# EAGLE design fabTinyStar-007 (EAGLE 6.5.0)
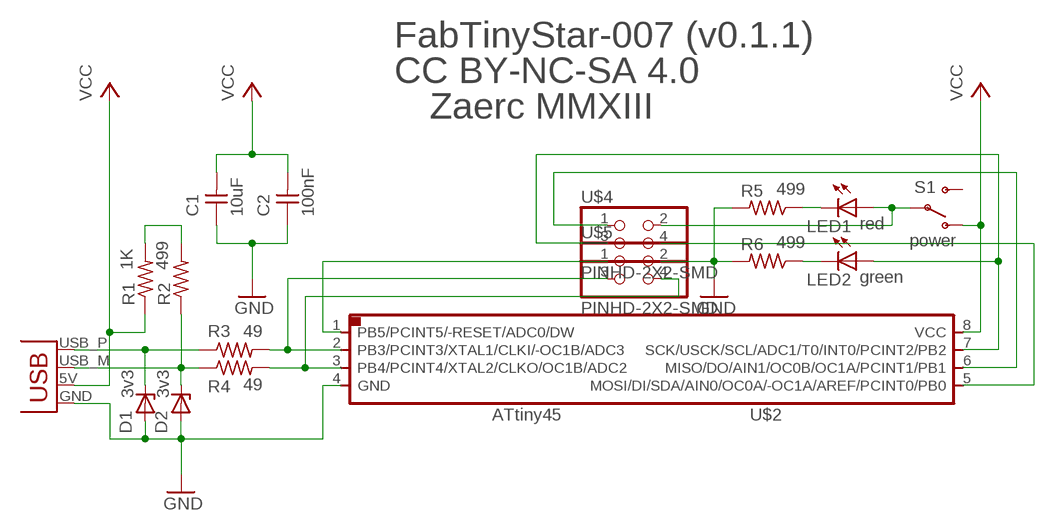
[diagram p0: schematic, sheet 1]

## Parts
C1  10uF  UNPOLARIZED_CAPACITOR1206  [1206]
C2  100nF  UNPOLARIZED_CAPACITOR1206  [1206]
D1  3v3  ZENER_DIODESOD123  [SOD123]
D2  3v3  ZENER_DIODESOD123  [SOD123]
LED1  red  LEDSMT1206  [1206]
LED2  green  LEDSMT1206  [1206]
R1  1K  RESISTOR1206  [1206]
R2  499  RESISTOR1206  [1206]
R3  49  RESISTOR1206  [1206]
R4  49  RESISTOR1206  [1206]
R5  499  RESISTOR1206  [1206]
R6  499  RESISTOR1206  [1206]
S1  power  SWITCH-SPSTSMD2  [SWITCH-SPDT-SMD]
U$1  USBPCB  [USB-A-PCB]
U$2  ATTINY45SI  [SOIC8]
U$4  PINHD-2X2-SMD  [2X02SMD]
U$5  PINHD-2X2-SMD  [2X02SMD]

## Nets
GND: C1.1 C2.1 D1.ANODE D2.ANODE R5.2 R6.2 U$1.GND U$2.4(GND) U$5.2
MISO: U$2.6(MISO/DO/AIN1/OC0B/OC1A/PCINT1/PB1) U$4.1
MOSI: U$2.5(MOSI/DI/SDA/AIN0/OC0A/-OC1A/AREF/PCINT0/PB0) U$4.4
N$1: R1.2 R2.2
N$2: R4.2 U$2.3(PB4/PCINT4/XTAL2/CLKO/OC1B/ADC2) U$5.4
N$3: D1.CATHODE R3.1 U$1.USB_P(D+)
N$4: R3.2 U$2.2(PB3/PCINT3/XTAL1/CLKI/-OC1B/ADC3) U$5.3
N$5: D2.CATHODE R2.1 R4.1 U$1.USB_M(D-)
N$13: LED2.C R6.1
N$14: LED1.C R5.1
RST: U$2.1(PB5/PCINT5/-RESET/ADC0/DW) U$5.1
SCK: LED2.A U$2.7(SCK/USCK/SCL/ADC1/T0/INT0/PCINT2/PB2) U$4.3
TVCC: LED1.A S1.2(P) U$4.2
VCC: C1.2 C2.2 R1.1 S1.1(O) U$1.5V(VBUS) U$2.8(VCC)
Unconnected: S1.3(S)

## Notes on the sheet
- FabTinyStar-007 (v0.1.1)
- CC BY-NC-SA 4.0
- Zaerc MMXIII

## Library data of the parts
C1 C2 = 01_FAB_Hello:UNPOLARIZED_CAPACITOR: unpolarized_capacitor
D1 D2 = 01_fab:ZENER_DIODE: zener diode
LED1 LED2 = led:LED: LED
R1-R6 = 01_FAB_Hello:RESISTOR
S1 = SparkFun:SWITCH-SPST: SPST Switch Simple slide switch. Spark Fun Electronics SKU : COM-00102
U$1 = SparkFun:USB: USB Connectors USB-B-PTH is fully proven SKU : PRT-00139 USB-miniB is fully proven SKU : PRT-00587 USB-A-PCB is untested. USB-A-H is throughly reviewed, but untested. Spark Fun Electronics SKU : PRT-00437 USB-B-SMT is throughly reviewed, but untested. Needs silkscreen touching up. USB-A-S has not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
U$2 = 01_fab:ATTINY45
U$4 U$5 = 01_fab:PINHD-2X2-SMD

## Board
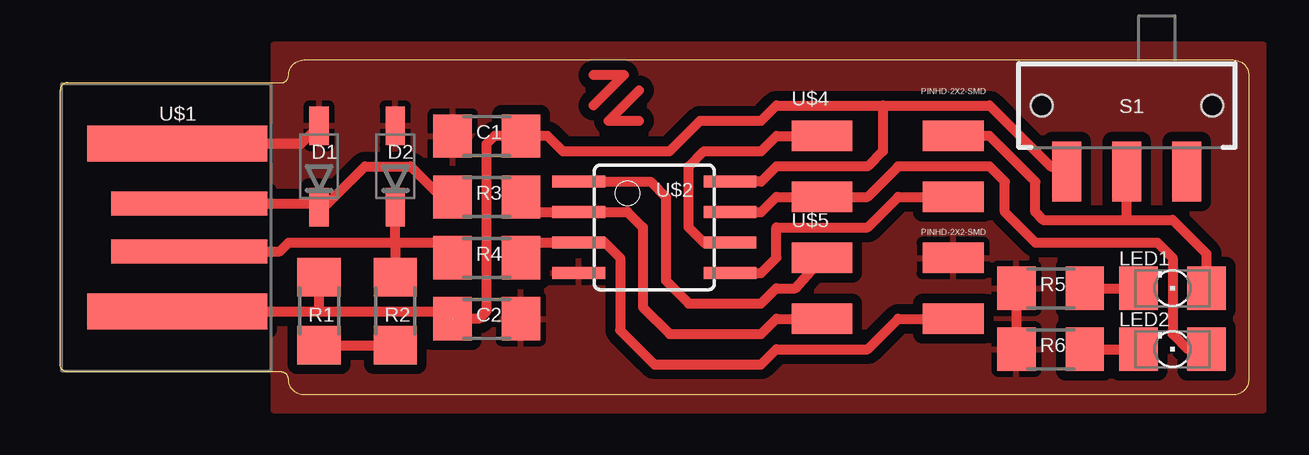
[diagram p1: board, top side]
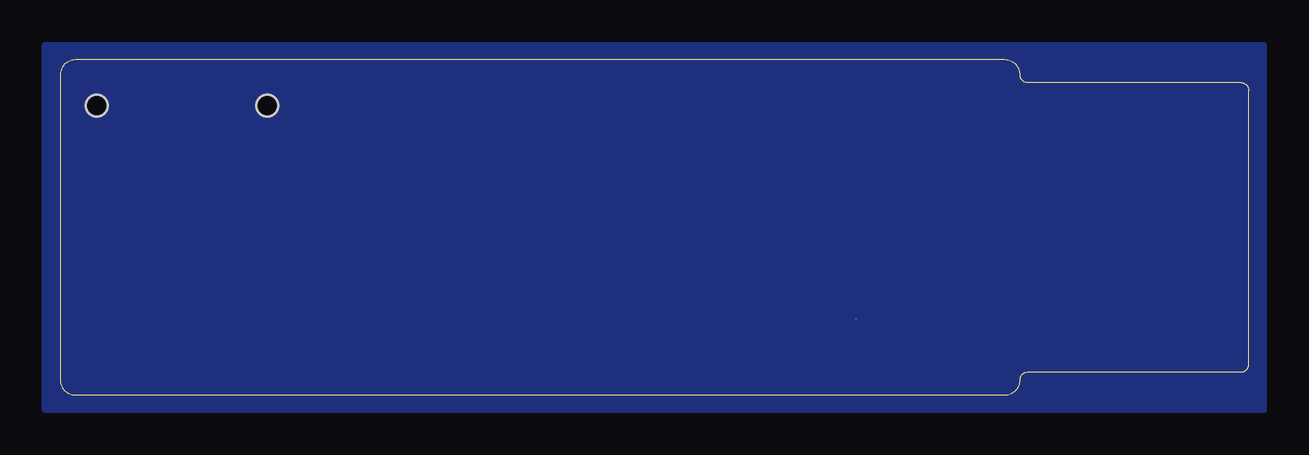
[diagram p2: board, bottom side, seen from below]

Size 49.53 x 13.97 mm. Coordinates in mm from the lower left corner, seen from the top.
Outline: 9.21,13.02 arc90 9.53,13.34 arc-90 10.16,13.97 48.9,13.97 arc-90 49.53,13.34 49.53,0.64 arc-90 48.9,0 10.16,0 arc-90 9.53,0.64 arc90 9.21,0.95 0.32,0.95 arc-90 0,1.27 0,12.7 arc-90 0.32,13.02 9.21,13.02
Copper layers (1*16): Top 0.035mm / dielectric 1.5mm / Bottom 0.035mm
Design rules "default *": minimum track width 10mil, minimum drill 24mil, track to track 16mil, track to pad 16mil, pad to pad 16mil, via to via 16mil, smd to smd 8mil, copper to edge 0mil, drill to drill 8mil, minimum pad ring 10mil, minimum via ring 8mil, stop-mask expansion 4mil, vias tented up to drill 0mil, thermal gap 10mil

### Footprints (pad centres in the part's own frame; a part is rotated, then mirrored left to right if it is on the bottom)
1206 = smd 1.6 x 1.803: 1 -1.422,0; 2 1.422,0
SOD123 = smd 1.6 x 0.8: ANODE 1.7,0; CATHODE -1.7,0
1206' = smd 1.6 x 1.803: A -1.422,0; C 1.422,0
SWITCH-SPDT-SMD = smd 1.2 x 2.5: 1 -2.5,-2.75; 2 0,-2.75; 3 2.5,-2.75 | hole 0.9: -3.55,0; 3.55,0
USB-A-PCB = smd 7.5 x 1.5: 5V -0.2,-3.5; GND -0.2,3.5 | smd 6.5 x 1: USB_M 0.3,-1; USB_P 0.3,1
SOIC8 = smd 0.5 x 2.2: 1 -1.905,-3.154; 2 -0.645,-3.154; 3 0.625,-3.154; 4 1.895,-3.154; 5 1.905,3.154; 6 0.635,3.154; 7 -0.635,3.154; 8 -1.905,3.154
2X02SMD = smd 2.54 x 1.27: 1 -2.54,1.27; 2 2.92,1.27; 3 -2.54,-1.27; 4 2.92,-1.27

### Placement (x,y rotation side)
C1  17.78,10.79 0 top
C2  17.78,3.17 180 top
D1  10.79,9.53 90 top
D2  13.97,9.53 90 top
LED1  red  [1206']  46.35,4.45 180 top
LED2  green  [1206']  46.35,1.91 180 top
R1  10.79,3.49 270 top
R2  13.97,3.49 270 top
R3  17.78,8.26 0 top
R4  17.78,5.71 0 top
R5  41.27,4.45 180 top
R6  41.27,1.91 180 top
S1  44.45,12.06 0 top
U$1  5.08,6.99 0 top
U$2  24.77,6.99 270 top
U$4  34.29,9.53 0 top
U$5  34.29,4.45 0 top

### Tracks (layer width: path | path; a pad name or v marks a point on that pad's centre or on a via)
GND
  Top 0.406: R5.2 R6.2 | U$1.GND 10.05,10.48 D1.ANODE
  pour Top: 8.89,-0.64 50.16,-0.64 50.16,14.61 8.89,14.61
MISO
  Top 0.406: U$2.6 26.83,6.35 26.19,6.99 26.19,9.53 26.83,10.16 29.21,10.16 29.84,10.79 U$4.1
MOSI
  Top 0.406: U$4.4 34.92,8.26 33.66,6.99 29.84,6.99 29.84,5.71 29.21,5.08 U$2.5
N$1
  Top 0.406: R1.2 R2.2
N$2
  Top 0.406: R4.2 19.85,6.36 U$2.3 22.69,6.36 23.34,5.71 23.34,2.7 24.77,1.27 29.21,1.27 29.84,1.91 33.66,1.91 34.92,3.17 U$5.4
N$3
  Top 0.406: U$1.USB_P 10.63,7.99 D1.CATHODE 11,7.83 12.7,9.53 14.61,9.53 15.88,8.26 R3.1
N$4
  Top 0.406: R3.2 19.83,7.63 U$2.2 23.64,7.63 24.29,6.99 24.29,3.65 25.4,2.54 29.21,2.54 29.84,3.17 U$5.3
N$5
  Top 0.406: 13.97,6.35 D2.CATHODE | U$1.USB_M 9.16,5.99 9.53,6.35 13.97,6.35 | 13.97,6.35 R2.1 | 13.97,6.35 15.72,6.35 R4.1
N$13
  Top 0.406: R6.1 LED2.C
N$14
  Top 0.406: R5.1 LED1.C
N$15
  pour Bottom: -0.64,-0.64 50.16,-0.64 50.16,14.61 -0.64,14.61
N$16
  Top 0.406: 22.23,13.34 23.5,13.34 22.23,12.06
N$17
  Top 0.406: 24.13,12.7 22.86,11.43 24.13,11.43
RST
  Top 0.406: U$2.1 24.61,8.89 25.24,8.26 25.24,4.76 26.19,3.81 29.21,3.81 29.84,4.45 30.64,4.45 U$5.1
SCK
  Top 0.406: U$2.7 29.21,7.62 29.84,8.26 U$4.3 33.66,8.26 34.92,9.53 38.73,9.53 39.37,8.89 39.37,7.62 40.64,6.35 45.72,6.35 46.35,5.71 46.35,2.54 46.99,1.91 LED2.A
TVCC
  Top 0.406: 44.45,7.3 46.35,7.3 47.78,5.88 LED1.A | 44.45,7.3 S1.2 | 44.45,7.3 40.96,7.3 40.64,7.62 40.64,8.89 38.73,10.79 U$4.2
VCC  (1 unrouted)
  Top 0.406: 34.29,12.06 34.29,10.16 33.66,9.53 29.84,9.53 29.21,8.89 U$2.8 | U$1.5V 10.79,3.48 | 10.79,3.48 R1.1 | 10.79,3.48 16.07,3.48 16.38,3.17 17.46,3.17 17.78,3.49 17.78,10.48 18.1,10.79 C1.2 20.32,10.79 20.95,10.16 25.4,10.16 26.67,11.43 29.21,11.43 29.84,12.06 34.29,12.06 | 34.29,12.06 38.73,12.06 41.27,9.53 41.74,9.53 S1.1

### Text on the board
tDocu: FabTinyStar v0.1.1 | CC BY-NC-SA 4.0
